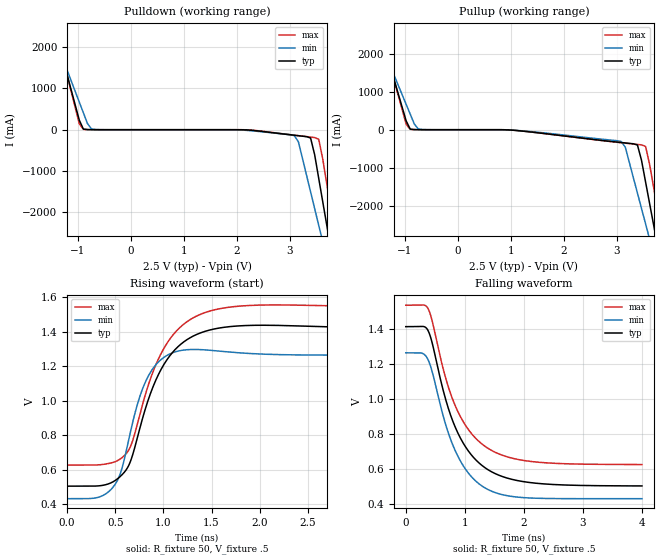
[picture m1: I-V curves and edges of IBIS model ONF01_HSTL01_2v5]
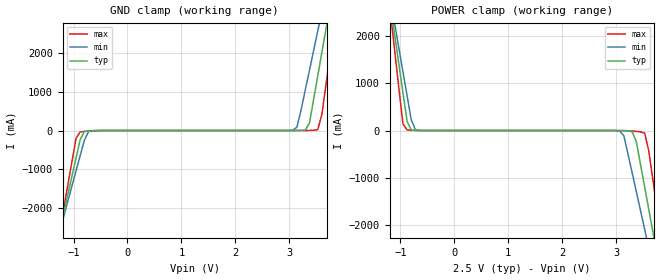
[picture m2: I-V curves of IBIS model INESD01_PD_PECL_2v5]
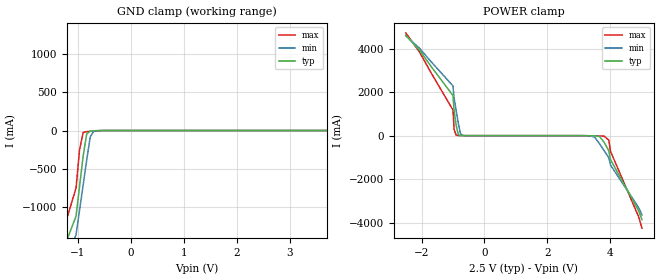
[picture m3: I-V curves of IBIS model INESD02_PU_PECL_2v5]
|   This file is an IBIS representation of the   |
|   Integrated Devices Technology, Inc.   |
|   ICS85314I01   |
|   Low Skew 1 to 5 LVPECL  Clock Buffer   |
[IBIS Ver]   4.1
[File name]   85314i_01.ibs
[File Rev]   0.1
[Date]   19 Mar 2009 | Last modified
|   Dec 20 2006 | Generated
[Source]   Originated at Integrated Devices Technology, Inc.
[Disclaimer]
IDT hereby grants the user of this IBIS model a non-exclusive,
nontransferable license to use this IBIS model under the following terms.
Before using this IBIS model, the user should read this license.
If the user does not accept these terms,  the IBIS model should be
returned to IDT within 30 days.
   The user is granted this license only to use the IBIS model and
is not granted rights to sell, load, rent, lease or license the IBIS
model in whole or in part, or in modified form to anyone other than
user. User may modify the IBIS model to suit its specific
applications but rights to derivative works and such modifications
shall belong to IDT.
   This IBIS model is provided on an "AS IS" basis and IDT makes
absolutely no warranty with respect to the information contained
herein. IDT DISCLAIMS AND CUSTOMER WAIVES ALL WARRANTIES, EXPRESS
OR IMPLIED, INCLUDING WARRANTIES OF MERCHANTABILITY OR FITNESS FOR
A PARTICULAR PURPOSE. The entire risk as to quality and performance
is with the Customer. ACCORDINGLY, IN NO EVENT SHALL THE COMPANY BE
LIABLE FOR ANY DAMAGES, WHETHER IN CONTRACT OR TORT,INCLUDING ANY
LOST PROFITS OR OTHER INCIDENTAL, CONSEQUENTIAL, EXEMPLARY, OR
PUNITIVE DAMAGES ARISING OUT OF THE USE OR APPLICATION OF THE IBIS
model provided in this package. Further, IDT reserves the right to
make changes without notice to any product herein to improve
reliability, function, or design. IDT does not convey any license
under patent rights or any other intellectual property rights,
including those of third parties.
   IDT is not obligated to provide maintenance or support
for the licensed IBIS model.
[Copyright]   Copyright 2003 by Integrated Devices Technology, Inc.
[Component]   ICS85314AGI-01
[Manufacturer] Integrated Devices Technology, Inc.
[Package]
|TSSOP 20 Lead
|   typ   min   max
R_pkg   51.85m   41.1m   62.6m
L_pkg   1.568nH   0.734nH   2.401nH
C_pkg   0.221pF   0.068pF   0.373pF
[Pin]   signal_name   model_name   R_pin   L_pin   C_pin
1   Q0   ONF01_HSTL01   62.6m   2.401n   0.373p
2   nQ0   ONF01_HSTL01   57.23m   1.985n   0.297p
3   Q1   ONF01_HSTL01   51.85m   1.568n   0.221p
4   nQ1   ONF01_HSTL01   46.78m   1.151n   0.145p
5   Q2   ONF01_HSTL01   41.1m   0.734n   0.068p
6   nQ2   ONF01_HSTL01   41.1m   0.734n   0.068p
7   Q3   ONF01_HSTL01   46.78m   1.151n   0.145p
8   nQ3   ONF01_HSTL01   51.85m   1.568n   0.221p
9   Q4   ONF01_HSTL01   57.23m   1.985n   0.297p
10   nQ4   ONF01_HSTL01   62.6m   2.401n   0.373p
11   VEE   GND   62.6m   2.401n   0.373p
12   CLK_SEL   INESD01_PD_PECL   57.23m   1.985n   0.297p
13   NC   NC   51.85m   1.568n   0.221p
14   nCLK0   INESD02_PU_PECL   46.78m   1.151n   0.145p
15   CLK0   INESD02_PD_PECL   41.1m   0.734n   0.068p
16   CLK1   INESD02_PD_PECL   41.1m   0.734n   0.068p
17   NC   NC   46.78m   1.151n   0.145p
18   VCC   POWER   51.85m   1.568n   0.221p
19   nCLK_EN   INESD01_PD   57.23m   1.985n   0.297p
20   VCC   POWER   62.6m   2.401n   0.373p
[Diff Pin]  inv_pin  vdiff tdelay_typ tdelay_min  tdelay_max
1   2   NA   0  0  0
3   4   NA   0  0  0
5   6   NA   0  0  0
7   8   NA   0  0  0
9   10   NA   0  0  0
[Component]   ICS85314AMI-01
[Manufacturer] Integrated Devices Technology, Inc.
[Package]
|SOIC 20 Lead
|   typ   min   max
R_pkg   57.15m   45.4m   68.9m
L_pkg   4.051n   2.187n   5.914n
C_pkg   0.796p   0.419p   1.173p
[Pin]   signal_name   model_name   R_pin   L_pin   C_pin
1   Q0   ONF01_HSTL01   68.90m   5.914n   1.173p
2   nQ0   ONF01_HSTL01   63.02m   4.983n   0.985p
3   Q1   ONF01_HSTL01   57.15m   4.051n   0.796p
4   nQ1   ONF01_HSTL01   51.25m   3.119n   0.608p
5   Q2   ONF01_HSTL01   45.40m   2.187n   0.419p
6   nQ2   ONF01_HSTL01   45.40m   2.187n   0.419p
7   Q3   ONF01_HSTL01   51.25m   3.119n   0.608p
8   nQ3   ONF01_HSTL01   57.15m   4.051n   0.796p
9   Q4   ONF01_HSTL01   63.02m   4.983n   0.985p
10   nQ4   ONF01_HSTL01   68.90m   5.914n   1.173p
11   VEE   GND   68.90m   5.914n   1.173p
12   CLK_SEL   INESD01_PD_PECL   63.02m   4.983n   0.985p
13   NC   NC   57.15m   4.051n   0.796p
14   nCLK0   INESD02_PU_PECL   51.25m   3.119n   0.608p
15   CLK0   INESD02_PD_PECL   45.40m   2.187n   0.419p
16   CLK1   INESD02_PD_PECL   45.40m   2.187n   0.419p
17   NC   NC   51.25m   3.119n   0.608p
18   VCC   POWER   57.15m   4.051n   0.796p
19   nCLK_EN   INESD01_PD   63.02m   4.983n   0.985p
20   VCC   POWER   68.90m   5.914n   1.173p
[Diff Pin]  inv_pin  vdiff tdelay_typ tdelay_min  tdelay_max
1   2   NA   0  0  0
3   4   NA   0  0  0
5   6   NA   0  0  0
7   8   NA   0  0  0
9   10   NA   0  0  0
[Model Selector] ONF01_HSTL01
ONF01_HSTL01_2v5  Buffer selection for 2v5
ONF01_HSTL01_3v3  Buffer selection for 3v3
[Model Selector] INESD01_PD_PECL
INESD01_PD_PECL_2v5  Buffer selection for 2v5
INESD01_PD_PECL_3v3  Buffer selection for 3v3
[Model Selector] INESD02_PU_PECL
INESD02_PU_PECL_2v5  Buffer selection for 2v5
INESD02_PU_PECL_3v3  Buffer selection for 3v3
[Model Selector] INESD02_PD_PECL
INESD02_PD_PECL_2v5  Buffer selection for 2v5
INESD02_PD_PECL_3v3  Buffer selection for 3v3
[Model Selector] INESD01_PD
INESD01_PD_2v5  Buffer selection for 2v5
INESD01_PD_3v3  Buffer selection for 3v3
| Models and submodels in the file (10): ONF01_HSTL01_2v5 (Output_ECL), INESD01_PD_PECL_2v5 (Input), INESD02_PU_PECL_2v5 (Input), INESD02_PD_PECL_2v5 (Input), INESD01_PD_2v5 (Input), ONF01_HSTL01_3v3 (Output_ECL), INESD01_PD_PECL_3v3 (Input), INESD02_PU_PECL_3v3 (Input), INESD02_PD_PECL_3v3 (Input), INESD01_PD_3v3 (Input)
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[Model] ONF01_HSTL01_2v5
Model_type  Output_ECL
Polarity   Non-Inverting
Vmeas = .89
Rref = 50
Cref = 0
Vref = .5
|Variable  typ   min   max
C_comp   2p   1.5p   2.5p
[Voltage Range]   2.5   2.375   2.625
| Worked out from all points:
|   rising waveform, R_fixture 50, V_fixture .5: 20-80 % time 350ps typ, 240ps min, 362ps max; typ from 0.504 V to 1.42 V
|   falling waveform, R_fixture 50, V_fixture .5: 20-80 % time 591ps typ, 523ps min, 591ps max; typ from 1.41 V to 0.504 V
| Open source, no load
|  Voltage   I(typ)   I(min)   I(max)
[Pullup]
-2.5V     7.585A     5.853A     7.966A
-1.582V   3.168A     2.738A     3.268A
-1.505V   2.8A       2.478A     2.877A
-892.9mV  15.1mA     409.7mA    8.262mA
-739.8mV  1.385mA    17.35mA    1.003mA
3.087V    -338.1mA   -312.6mA   -343.9mA
3.393V    -404.5mA   -1.675A    -388.5mA
3.469V    -807.4mA   -2.079A    -400mA
3.546V    -1.379A    -2.483A    -441.2mA
3.699V    -2.523A    -3.292A    -1.528A
3.852V    -3.666A    -4.1A      -2.744A
5V        -12.24A    -10.16A    -11.86A
[Pulldown]
-2.5V     7.585A     5.853A     7.966A
-1.505V   2.8A       2.478A     2.877A
-1.429V   2.433A     2.219A     2.485A
-892.9mV  15.1mA     409.7mA    8.262mA
-663.3mV  413.9uA    3.764mA    253.1uA
3.087V    -134.5mA   -144.5mA   -132.9mA
3.393V    -201.7mA   -1.506A    -178.4mA
3.469V    -604.8mA   -1.91A     -190.2mA
3.546V    -1.177A    -2.315A    -231.7mA
3.699V    -2.321A    -3.123A    -1.319A
3.852V    -3.464A    -3.931A    -2.535A
5V        -12.04A    -9.99A     -11.65A
[Ramp]
|   typ   min   max
dV/dt_r   0.747/0.607n   0.692/0.422n   0.743/0.611n
dV/dt_f   0.728/0.954n   0.666/0.82n   0.729/0.951n
R_load =   50.0000
[Rising Waveform]
R_fixture = 50
V_fixture = .5   | VCC_typ - 2V
V_fixture_max = 0.625   | VCC_max - 2V
V_fixture_min = 0.375   | VCC_min - 2V
C_fixture = 0.0p
| Time   typ   min   max
0s        503.5mV    430.9mV    625.7mV
426.4ps   516.2mV    469mV      634.6mV
537.1ps   552.3mV    553.7mV    655.9mV
615ps     599.4mV    709mV      693.2mV
725.7ps   775.8mV    969.5mV    854.9mV
824.1ps   972.5mV    1.121V     1.055V
1.099ns   1.282V     1.278V     1.38V
1.365ns   1.389V     1.296V     1.496V
1.755ns   1.433V     1.279V     1.547V
3.997ns   1.415V     1.264V     1.538V
[Falling Waveform]
R_fixture = 50
V_fixture = .5   | VCC_typ - 2V
V_fixture_max = 0.625   | VCC_max - 2V
V_fixture_min = 0.375   | VCC_min - 2V
C_fixture = 0.0p
| Time   typ   min   max
0s        1.413V     1.264V     1.536V
270.6ps   1.415V     1.262V     1.537V
373.1ps   1.394V     1.228V     1.519V
446.9ps   1.321V     1.157V     1.446V
668.3ps   1.006V     861.8mV    1.129V
832.3ps   843.5mV    708.9mV    965.8mV
1.074ns   696.6mV    571.2mV    819.3mV
1.365ns   602.2mV    488mV      724.4mV
2.148ns   521.3mV    434.3mV    642.4mV
3.997ns   503.9mV    431mV      626mV
[Model] INESD01_PD_PECL_2v5
Model_type  Input
Polarity   Non-Inverting
Vinl = 0.9
Vinh = 1.6V
|   typ   min   max
C_comp   2pF   1.5pF   2.5pF
|   typ   min   max
[Voltage range]  2.5V   2.375V   2.625V
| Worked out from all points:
|   GND clamp passes 1 mA (typ) near -0.55 V on its own axis
|   POWER clamp passes 1 mA (typ) near -0.67 V on its own axis
[GND_clamp]
|Voltage   I(typ)   I(min)   I(max)
-2.5V     -10.33A    -9.044A    -12.47A
-1.263V   -2.632A    -2.639A    -2.655A
-953.6mV  -711.7mA   -1.044A    -200.4mA
-876.3mV  -232.7mA   -645.9mA   -36.86mA
-644.3mV  -3.696mA   -3.384mA   -8.124mA
3.067V    149.4uA    7.715mA    47.92uA
3.144V    502.3uA    86.83mA    64.06uA
3.376V    191.2mA    1.558A     2.431mA
3.531V    1.419A     2.581A     23.33mA
3.686V    2.649A     3.605A     1.215A
3.84V     3.882A     4.631A     2.791A
5V        13.16A     12.34A     14.65A
[POWER_clamp]
|Voltage   I(typ)   I(min)   I(max)
-2.5V     13.16A     11.51A     15.93A
-1.186V   2.649A     2.777A     2.489A
-1.108V   2.034A     2.265A     1.701A
-953.6mV  804mA      1.243A     144.3mA
-876.3mV  191.2mA    733.1mA    11.85mA
-644.3mV  502.3uA    1.889mA    389.3uA
3.067V    -1.226mA   -11.24mA   -226.8uA
3.299V    -24.5mA    -891.1mA   -10.73mA
3.531V    -1.191A    -2.086A    -51.9mA
3.686V    -2.151A    -2.885A    -1.049A
3.84V     -3.112A    -3.684A    -2.276A
5V        -10.33A    -9.692A    -11.48A
[Model] INESD02_PU_PECL_2v5
Model_type   Input
Polarity   Non-Inverting
Vinl = .8V
Vinh =  2V
|   typ   min   max
C_comp   2pF   1.5pF   2.5pF
|   typ   min   max
[Voltage range]  2.5V   2.375V   2.625V
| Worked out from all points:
|   GND clamp passes 1 mA (typ) near -0.59 V on its own axis
|   POWER clamp passes 1 mA (typ) near -0.70 V on its own axis
[GND_clamp]
|Voltage   I(typ)   I(min)   I(max)
-2.5V     -3.894A    -3.674A    -4.294A
-1.25V    -1.521A    -1.7A      -1.261A
-1.031V   -1.125A    -1.372A    -755.3mA
-896.9mV  -335.4mA   -714.7mA   -27.06mA
-695.9mV  -3.401mA   -10.7mA    -6.467mA
3.995V    711.6uA    10.32mA    481.3uA
4.062V    4.029mA    88.04mA    1.401mA
4.129V    40.44mA    547.3mA    3.341mA
4.196V    445.8mA    1.124A     14.79mA
4.263V    1.139A     1.7A       275.9mA
4.5V      1.832A     2.277A     1.163A
5V        3.219A     3.431A     2.937A
[POWER_clamp]
|Voltage   I(typ)   I(min)   I(max)
-2.5V     4.617A     4.594A     4.726A
-1V       1.842A     2.286A     1.176A
-963.9mV  1.149A     1.709A     289.6mA
-896.9mV  456.4mA    1.132A     15.33mA
-829.9mV  42.02mA    556.1mA    3.389mA
-762.9mV  4.159mA    91.01mA    1.421mA
-695.9mV  727.9uA    10.67mA    490.4uA
3.35V     -3.204mA   -9.193mA   -6.2mA
3.8V      -305mA     -689.5mA   -24.7mA
3.95V     -699.9mA   -1.018A    -211mA
4V        -1.095A    -1.346A    -716.4mA
5V        -3.863A    -3.649A    -4.255A
